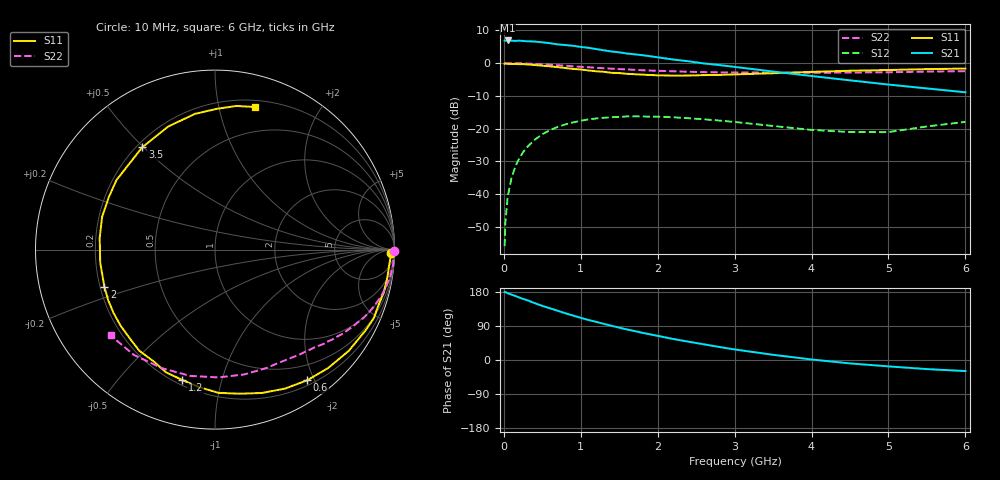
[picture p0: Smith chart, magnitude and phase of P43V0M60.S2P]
! SIEMENS Small Signal Semiconductors
! BFP182
! Si NPN RF Bipolar Junction Transistor in SOT143
! VCE = 3 V  IC = 0.6 mA
! Common Emitter S-Parameters:  March  1996
# GHz  S  MA  R  50
!  f  S11  S21  S12  S22
! GHz  MAG  ANG  MAG  ANG  MAG  ANG  MAG  ANG
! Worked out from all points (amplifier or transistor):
!   36 points, 10 MHz to 6 GHz, reference 50 ohm
!   highest |S21| = 6.9 dB at 50 MHz (marker M1)
!   |S21| within 3 dB of that: start of sweep to 1.297 GHz
!   unconditionally stable (mu >= 1): 2.887 GHz to end of sweep
!   at 250 MHz: K = 0.09, MSG = 17.0 dB, |S12| = -27.2 dB
!   at 1.4 GHz: K = 0.50, MSG = 10.0 dB, |S12| = -16.5 dB
!   at 6 GHz: K = 1.17, MAG = 2.0 dB, |S12| = -18.0 dB
!   S11 on the Smith chart (normalised r, x): 10 MHz: 56, -45; 600 MHz: 0.27, -1.90; 1.2 GHz: 0.23, -0.76; 2 GHz: 0.22, -0.16; 3.5 GHz: 0.22, +0.50; 6 GHz: 0.26, +1.28
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0.01  0.9786 -1.0  2.202 179.6  0.0016 87.7  0.9993 -0.3
0.02  0.9804 -2.0  2.198 179.2  0.0037 88.6  0.9922 -0.6
0.05  0.9748 -4.8  2.216 176.2  0.0091 87.4  0.9986 -1.6
0.1  0.9726 -9.3  2.2 172.6  0.0177 83.1  0.9956 -3.4
0.15  0.9703 -14.3  2.178 168.9  0.0265 80.4  0.9963 -5.1
0.25  0.9641 -23.3  2.177 161.2  0.0435 75.2  0.9885 -8.5
0.4  0.9348 -37.1  2.133 150.1  0.0673 66.2  0.9717 -13.2
0.5  0.9126 -46.3  2.076 142.8  0.0819 60.2  0.958 -16.4
0.6  0.891 -54.8  2.012 136.4  0.0946 54.9  0.9422 -19.3
0.9  0.8148 -80.2  1.836 117.3  0.1244 40.1  0.8928 -27.0
1.1  0.7713 -96.6  1.712 105.6  0.1382 31.6  0.8623 -31.6
1.2  0.7493 -104.0  1.638 100.6  0.1427 27.2  0.8488 -33.8
1.6  0.6859 -133.7  1.4 80.6  0.1534 14.2  0.8012 -41.0
2  0.6503 -161.4  1.225 63.7  0.1519 3.8  0.7616 -47.8
2.2  0.6436 -173.5  1.134 55.5  0.1488 -0.9  0.7501 -51.4
2.8  0.66 153.6  0.933 34.4  0.1326 -10.5  0.7215 -62.2
3.5  0.6996 125.4  0.742 13.7  0.1096 -15.1  0.7145 -76.7
4  0.7337 110.8  0.635 1.4  0.0954 -11.1  0.7124 -88.6
4.5  0.7643 98.4  0.545 -9.0  0.0885 -3.6  0.7172 -101.3
5  0.784 89.4  0.47 -16.8  0.0884 9.2  0.7241 -114.3
5.5  0.809 81.6  0.41 -24.0  0.1078 14.7  0.7409 -127.7
6  0.8246 74.5  0.358 -29.2  0.1264 15.4  0.7529 -140.6
